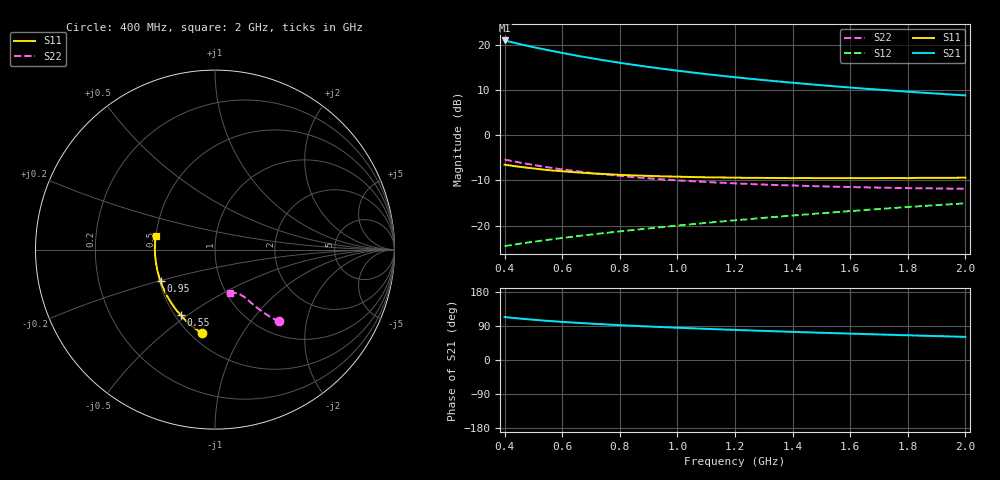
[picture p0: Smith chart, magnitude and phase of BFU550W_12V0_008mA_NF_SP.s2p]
! Filename:  P:\Prog\Test\Noise\ATS_data\Testdata_Net\06 Compressed Noise after Statistics\BFU550W_APM2013_11_D05_12p0V_008mA_NF_CM01_D.sf
! Date/Time: Tue 26/Mar/2013 16:25:26
! BFU550W_APM2013_11_D05_12p0V_1to35mA_NF_CM01_Bias5_R.sf
! Noise Parameter Data File
! BFU550W_APM2013_11_D05_12p0V_1to35mA_NF_CM01
! Date/time: Mon Mar 25 15:58:35 2013
! VAR V_out= 12.001000
! VAR I_out= 8.000000
! VAR V_in= 0.794900
! VAR I_in= 0.068405
! Device data file deembeded for feedlines and parallel
! Original file: \06 Compressed Noise after Statistics\BFU550W_APM2013_11_D05_12p0V_008mA_NF_CM01_R.sf
! Feed-files: PR019V01_070313_Feed1.s2p, PR019V01_070313_Feed2.s2p
! Parallel-file: PR019V01_070313_Par.s2p
# MHz S MA R 50
!  Freq-MHz  S11-mag  S11-arg  S21-mag  S21-arg  S12-mag  S12-arg  S22-mag  S22-arg
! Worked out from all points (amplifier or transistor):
!   37 points, 400 MHz to 2 GHz, reference 50 ohm
!   highest |S21| = 21.0 dB at 400 MHz (marker M1)
!   |S21| within 3 dB of that: start of sweep to 619.9 MHz
!   unconditionally stable (mu >= 1): 1.552 GHz to end of sweep
!   at 500 MHz: K = 0.66, MSG = 21.6 dB, |S12| = -23.6 dB
!   at 1.1 GHz: K = 0.94, MSG = 16.5 dB, |S12| = -19.4 dB
!   at 2 GHz: K = 1.01, MAG = 11.2 dB, |S12| = -15.1 dB
!   lowest NFmin = 0.70 dB at 400 MHz
!   S11 on the Smith chart (normalised r, x): 400 MHz: 0.57, -0.68; 550 MHz: 0.54, -0.47; 950 MHz: 0.51, -0.20; 2 GHz: 0.50, +0.08
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400  0.4722 -98.6  11.21 113.4  0.05909 56.3  0.5372 -48.1
420  0.4621 -101.6  10.82 111.8  0.06061 56.1  0.5222 -48.9
440  0.4527 -104.4  10.45 110.3  0.06204 55.9  0.5076 -49.5
460  0.4446 -107.0  10.1 108.9  0.06343 55.9  0.4939 -50.2
500  0.429 -112.1  9.455 106.3  0.06613 55.8  0.4688 -51.3
550  0.4114 -117.7  8.771 103.3  0.06948 56.0  0.4415 -52.4
600  0.3992 -123.1  8.16 100.6  0.07283 56.2  0.4181 -53.3
650  0.3878 -127.7  7.617 98.2  0.07612 56.5  0.3993 -54.1
700  0.3784 -132.2  7.144 95.9  0.07946 56.9  0.3822 -54.8
750  0.3716 -136.1  6.722 93.9  0.08278 57.2  0.3675 -55.4
800  0.3641 -140.1  6.348 92.0  0.08616 57.6  0.355 -56.0
850  0.359 -143.8  6.012 90.1  0.08952 58.0  0.3432 -56.4
950  0.3504 -150.0  5.438 86.8  0.09644 58.8  0.3246 -57.5
1050  0.3447 -155.8  4.964 83.7  0.1035 59.4  0.3098 -58.5
1150  0.3409 -161.2  4.566 80.8  0.1106 59.9  0.2982 -59.5
1200  0.3389 -163.4  4.394 79.4  0.1143 60.1  0.2933 -60.1
1250  0.3374 -166.0  4.23 78.1  0.1179 60.3  0.2884 -60.4
1350  0.3361 -170.1  3.944 75.5  0.1255 60.7  0.2806 -61.6
1500  0.3346 -176.1  3.581 71.9  0.1368 60.9  0.272 -63.6
1650  0.3348 178.4  3.283 68.5  0.1484 61.0  0.265 -65.6
1750  0.3358 175.2  3.116 66.3  0.1563 61.0  0.261 -67.1
2000  0.3392 167.6  2.763 61.0  0.1762 60.6  0.2551 -71.3
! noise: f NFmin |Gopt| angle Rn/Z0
400  0.6975  0.05958  86.89  0.0923
460  0.7252  0.07277  98.97  0.0869
600  0.7455  0.09446  94.61  0.0946
800  0.7702  0.1174  125.8  0.0833
1000  0.8057  0.1563  136.4  0.0763
1200  0.8349  0.1696  143.6  0.0782
1400  0.8756  0.2166  154.1  0.0663
1600  0.8833  0.2413  163.2  0.0646
1800  0.936  0.278  175.3  0.0592
2000  0.9266  0.2991  -172  0.0628
